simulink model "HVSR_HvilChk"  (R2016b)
settings: Solver=FixedStepDiscrete  StartTime=0.0  StopTime=10.0  FixedStep=0.02  RelTol=1e-3  EnableMultiTasking=on
undefined symbols (not defined in the file or in its folder): BCCR_cntHvilDiag_CW, bin2dec, HVSR_dcHvilPwmDutyHi_C, HVSR_dcHvilPwmDutyLo_C, HVSR_dcHvilPwmDutyNrm_C, HVSR_dcHvilPwmDutyOpl_C, HVSR_dcHvilPwmDutyOptSet_C, HVSR_dcHvilPwmDutyThres_C, HVSR_fHvilPwmFrqHi_C, HVSR_fHvilPwmFrqLo_C, HVSR_tiHvilOplErr_C, HVSR_tiHvilScbErr_C, HVSR_tiHvilScgErr_C, HVSR_uKL30ThresHi_C, HVSR_uKL30ThresLo_C
libraries: simulink x39

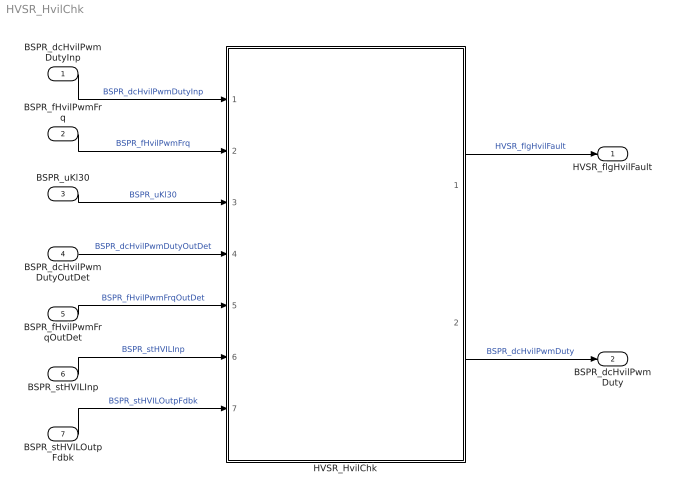
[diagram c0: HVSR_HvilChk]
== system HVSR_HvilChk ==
  BSPR_dcHvilPwmDutyInp : Inport
  BSPR_fHvilPwmFrq : Inport  Port=2
  BSPR_uKl30 : Inport  Port=3
  BSPR_dcHvilPwmDutyOutDet : Inport  Port=4
  BSPR_fHvilPwmFrqOutDet : Inport  Port=5
  BSPR_stHVILInp : Inport  Port=6
  BSPR_stHVILOutpFdbk : Inport  Port=7
  HVSR_HvilChk : Subsystem
  HVSR_flgHvilFault : Outport
  BSPR_dcHvilPwmDuty : Outport  Port=2
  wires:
  BSPR_uKl30/1 -> HVSR_HvilChk/3(BSPR_uKl30)  "BSPR_uKl30"
  BSPR_dcHvilPwmDutyInp/1 -> HVSR_HvilChk/1(BSPR_dcHvilPwmDutyInp)  "BSPR_dcHvilPwmDutyInp"
  HVSR_HvilChk/1(HVSR_flgHvilFault) -> HVSR_flgHvilFault/1  "HVSR_flgHvilFault"
  BSPR_fHvilPwmFrq/1 -> HVSR_HvilChk/2(BSPR_fHvilPwmFrq)  "BSPR_fHvilPwmFrq"
  BSPR_dcHvilPwmDutyOutDet/1 -> HVSR_HvilChk/4(BSPR_dcHvilPwmDutyOutDet)  "BSPR_dcHvilPwmDutyOutDet"
  BSPR_fHvilPwmFrqOutDet/1 -> HVSR_HvilChk/5(BSPR_fHvilPwmFrqOutDet)  "BSPR_fHvilPwmFrqOutDet"
  BSPR_stHVILInp/1 -> HVSR_HvilChk/6(BSPR_stHVILInp)  "BSPR_stHVILInp"
  BSPR_stHVILOutpFdbk/1 -> HVSR_HvilChk/7(BSPR_stHVILOutpFdbk)  "BSPR_stHVILOutpFdbk"
  HVSR_HvilChk/2(BSPR_dcHvilPwmDuty) -> BSPR_dcHvilPwmDuty/1  "BSPR_dcHvilPwmDuty"

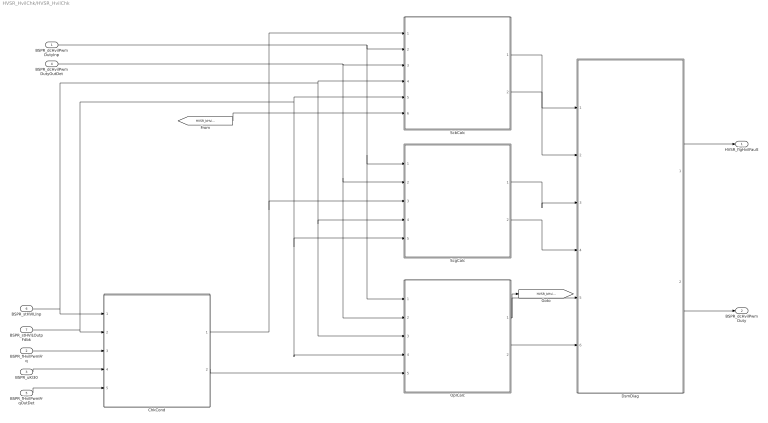
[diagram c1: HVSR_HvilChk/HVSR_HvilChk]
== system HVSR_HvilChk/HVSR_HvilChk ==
  BSPR_dcHvilPwmDutyInp : Inport
  BSPR_fHvilPwmFrq : Inport  Port=2
  BSPR_uKl30 : Inport  Port=3
  BSPR_dcHvilPwmDutyOutDet : Inport  Port=4
  BSPR_fHvilPwmFrqOutDet : Inport  Port=5
  BSPR_stHVILInp : Inport  Port=6
  BSPR_stHVILOutpFdbk : Inport  Port=7
  ChkCond : Subsystem
  DsmDiag : Subsystem
  OplCalc : Subsystem
  ScbCalc : Subsystem
  ScgCalc : Subsystem
  HVSR_flgHvilFault : Outport
  BSPR_dcHvilPwmDuty : Outport  Port=2
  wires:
  BSPR_uKl30/1 -> ChkCond/4(BSPR_uKl30)
  BSPR_dcHvilPwmDutyInp/1 -> ScgCalc/1(BSPR_dcHvilPwmDutyInp), OplCalc/1(BSPR_dcHvilPwmDutyInp), ScbCalc/2(BSPR_dcHvilPwmDutyInp)
  ScgCalc/1(HVSR_bHvilScgErrDet) -> DsmDiag/3(HVSR_bHvilScgErrDet)
  ScgCalc/2(HVSR_bHvilScgErrHeal) -> DsmDiag/4(HVSR_bHvilScgErrHeal)
  ChkCond/1(BSPR_bKl30HvilDiagCond) -> ScbCalc/1(BSPR_bKl30HvilDiagCond), ScgCalc/3(BSPR_bKl30HvilDiagCond)
  ScbCalc/1(HVSR_bHvilScbErrDet) -> DsmDiag/1(HVSR_bHvilScbErrDet)
  ScbCalc/2(HVSR_bHvilScbErrHeal) -> DsmDiag/2(HVSR_bHvilScbErrHeal)
  DsmDiag/1(HVSR_flgHvilFault) -> HVSR_flgHvilFault/1
  OplCalc/2(HVSR_bHvilOplErrHeal) -> DsmDiag/6(HVSR_bHvilOplErrHeal)
  OplCalc/1(HVSR_bHvilOplErrDet) -> [HVSR_bHvilOplErrDet], DsmDiag/5(HVSR_bHvilOplErrDet)
  BSPR_fHvilPwmFrq/1 -> ChkCond/3(BSPR_fHvilPwmFrq)
  ChkCond/2(BSPR_bHvilDiagCond) -> OplCalc/5(BSPR_bHvilDiagCond)
  BSPR_dcHvilPwmDutyOutDet/1 -> ScgCalc/2(BSPR_dcHvilPwmDutyOutDet), OplCalc/2(BSPR_dcHvilPwmDutyOutDet), ScbCalc/3(BSPR_dcHvilPwmDutyOutDet)
  BSPR_fHvilPwmFrqOutDet/1 -> ChkCond/5(BSPR_fHvilPwmFrqOutDet)
  BSPR_stHVILInp/1 -> ChkCond/1(BSPR_stHVILInp), ScgCalc/4(BSPR_stHVILInp), OplCalc/3(BSPR_stHVILInp), ScbCalc/4(BSPR_stHVILInp)
  BSPR_stHVILOutpFdbk/1 -> ChkCond/2(BSPR_stHVILOutpFdbk), ScgCalc/5(BSPR_stHVILOutpFdbk), OplCalc/4(BSPR_stHVILOutpFdbk), ScbCalc/5(BSPR_stHVILOutpFdbk)
  DsmDiag/2(BSPR_dcHvilPwmDuty) -> BSPR_dcHvilPwmDuty/1
  [HVSR_bHvilOplErrDet] -> ScbCalc/6(HVSR_bHvilOplErrDet)

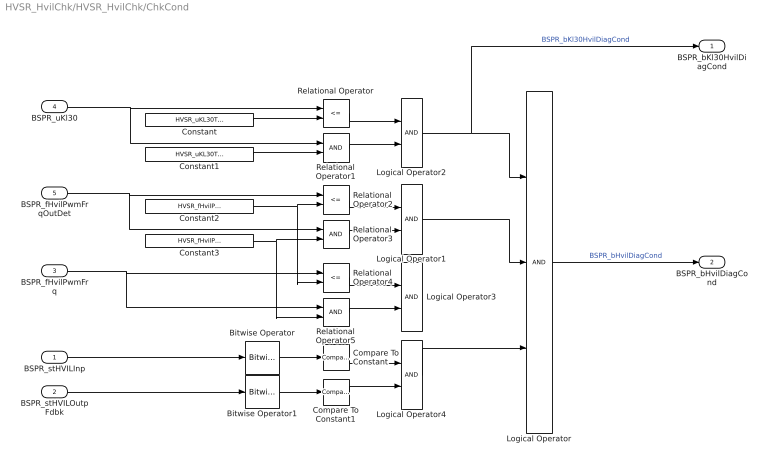
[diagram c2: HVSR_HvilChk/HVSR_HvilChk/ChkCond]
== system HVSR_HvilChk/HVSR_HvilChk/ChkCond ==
  BSPR_stHVILInp : Inport
  BSPR_stHVILOutpFdbk : Inport  Port=2
  BSPR_fHvilPwmFrq : Inport  Port=3
  BSPR_uKl30 : Inport  Port=4
  BSPR_fHvilPwmFrqOutDet : Inport  Port=5
  Bitwise Operator : simulink/Logic and Bit Operations/Bitwise Operator  logicop=AND  UseBitMask=on  BitMask=bin2dec('00010000')  BitMaskRealWorld=Stored Integer
  Bitwise Operator1 : simulink/Logic and Bit Operations/Bitwise Operator  logicop=AND  UseBitMask=on  BitMask=bin2dec('00010000')  BitMaskRealWorld=Stored Integer
  Compare To Constant : simulink/Logic and Bit Operations/Compare To Constant  relop===  const=0  OutDataTypeStr=boolean
  Compare To Constant1 : simulink/Logic and Bit Operations/Compare To Constant  relop===  const=0  OutDataTypeStr=boolean
  Constant : Constant  Value=HVSR_uKL30ThresHi_C
  Constant1 : Constant  Value=HVSR_uKL30ThresLo_C
  Constant2 : Constant  Value=HVSR_fHvilPwmFrqHi_C
  Constant3 : Constant  Value=HVSR_fHvilPwmFrqLo_C
  Logical Operator : Logic  Inputs=3  AllPortsSameDT=off  OutDataTypeStr=boolean
  Logical Operator1 : Logic  AllPortsSameDT=off  OutDataTypeStr=boolean
  Logical Operator2 : Logic  AllPortsSameDT=off  OutDataTypeStr=boolean
  Logical Operator3 : Logic  Commented=on  AllPortsSameDT=off  OutDataTypeStr=boolean
  Logical Operator4 : Logic  AllPortsSameDT=off  OutDataTypeStr=boolean
  Relational Operator : RelationalOperator  Operator=<=  OutDataTypeStr=boolean  RndMeth=Simplest
  Relational Operator1 : RelationalOperator  OutDataTypeStr=boolean  RndMeth=Simplest
  Relational Operator2 : RelationalOperator  Operator=<=  OutDataTypeStr=boolean  RndMeth=Simplest
  Relational Operator3 : RelationalOperator  OutDataTypeStr=boolean  RndMeth=Simplest
  Relational Operator4 : RelationalOperator  Commented=on  Operator=<=  OutDataTypeStr=boolean  RndMeth=Simplest
  Relational Operator5 : RelationalOperator  Commented=on  OutDataTypeStr=boolean  RndMeth=Simplest
  BSPR_bKl30HvilDiagCond : Outport
  BSPR_bHvilDiagCond : Outport  Port=2
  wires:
  BSPR_uKl30/1 -> Relational Operator/1, Relational Operator1/1
  Logical Operator/1 -> BSPR_bHvilDiagCond/1  "BSPR_bHvilDiagCond"
  Constant/1 -> Relational Operator/2
  Constant1/1 -> Relational Operator1/2
  BSPR_fHvilPwmFrqOutDet/1 -> Relational Operator2/1, Relational Operator3/1
  Relational Operator/1 -> Logical Operator2/1
  Relational Operator1/1 -> Logical Operator2/2
  Logical Operator2/1 -> BSPR_bKl30HvilDiagCond/1, Logical Operator/1  "BSPR_bKl30HvilDiagCond"
  BSPR_fHvilPwmFrq/1 -> Relational Operator5/1, Relational Operator4/1
  Constant2/1 -> Relational Operator4/2, Relational Operator2/2
  Constant3/1 -> Relational Operator5/2, Relational Operator3/2
  Relational Operator4/1 -> Logical Operator3/1
  Relational Operator5/1 -> Logical Operator3/2
  Relational Operator2/1 -> Logical Operator1/1
  Relational Operator3/1 -> Logical Operator1/2
  Logical Operator1/1 -> Logical Operator/2
  Logical Operator3/1 -> ?
  BSPR_stHVILInp/1 -> Bitwise Operator/1
  BSPR_stHVILOutpFdbk/1 -> Bitwise Operator1/1
  Bitwise Operator/1 -> Compare To Constant/1
  Bitwise Operator1/1 -> Compare To Constant1/1
  Compare To Constant/1 -> Logical Operator4/1
  Compare To Constant1/1 -> Logical Operator4/2
  Logical Operator4/1 -> Logical Operator/3

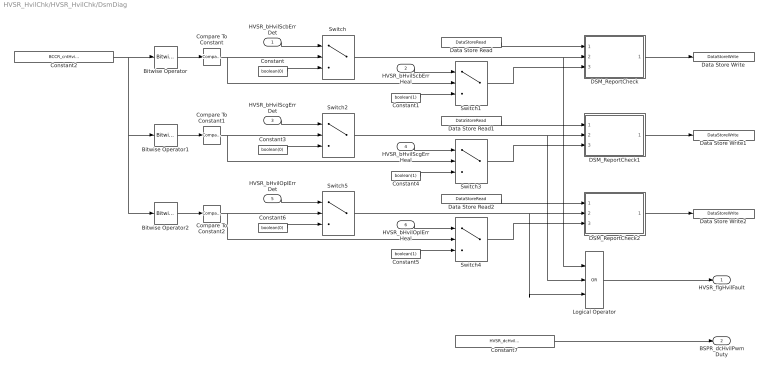
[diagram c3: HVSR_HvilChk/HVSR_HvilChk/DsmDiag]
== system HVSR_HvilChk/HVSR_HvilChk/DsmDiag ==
  HVSR_bHvilScbErrDet : Inport
  HVSR_bHvilScbErrHeal : Inport  Port=2
  HVSR_bHvilScgErrDet : Inport  Port=3
  HVSR_bHvilScgErrHeal : Inport  Port=4
  HVSR_bHvilOplErrDet : Inport  Port=5
  HVSR_bHvilOplErrHeal : Inport  Port=6
  Bitwise Operator : simulink/Logic and Bit Operations/Bitwise Operator  logicop=AND  UseBitMask=on  BitMask=bin2dec('00000001')  BitMaskRealWorld=Stored Integer
  Bitwise Operator1 : simulink/Logic and Bit Operations/Bitwise Operator  logicop=AND  UseBitMask=on  BitMask=bin2dec('00000010')  BitMaskRealWorld=Stored Integer
  Bitwise Operator2 : simulink/Logic and Bit Operations/Bitwise Operator  logicop=AND  UseBitMask=on  BitMask=bin2dec('00000100')  BitMaskRealWorld=Stored Integer
  Compare To Constant : simulink/Logic and Bit Operations/Compare To Constant  relop===  const=1  OutDataTypeStr=boolean
  Compare To Constant1 : simulink/Logic and Bit Operations/Compare To Constant  relop===  const=2  OutDataTypeStr=boolean
  Compare To Constant2 : simulink/Logic and Bit Operations/Compare To Constant  relop===  const=4  OutDataTypeStr=boolean
  Constant : Constant  Value=boolean(0)  OutDataTypeStr=boolean
  Constant1 : Constant  Value=boolean(1)  OutDataTypeStr=boolean
  Constant2 : Constant  Value=BCCR_cntHvilDiag_CW
  Constant3 : Constant  Value=boolean(0)  OutDataTypeStr=boolean
  Constant4 : Constant  Value=boolean(1)  OutDataTypeStr=boolean
  Constant5 : Constant  Value=boolean(1)  OutDataTypeStr=boolean
  Constant6 : Constant  Value=boolean(0)  OutDataTypeStr=boolean
  Constant7 : Constant  Value=HVSR_dcHvilPwmDutyOptSet_C
  DSM_ReportCheck : Subsystem  TreatAsAtomicUnit=on  RTWFcnName=DSM_ReportCheck  RTWFileName=SrvLib
  DSM_ReportCheck1 : Subsystem  TreatAsAtomicUnit=on  RTWFcnName=DSM_ReportCheck  RTWFileName=SrvLib
  DSM_ReportCheck2 : Subsystem  TreatAsAtomicUnit=on  RTWFcnName=DSM_ReportCheck  RTWFileName=SrvLib
  Data Store Read : DataStoreRead  DataStoreName=DFC_HvilMax
  Data Store Read1 : DataStoreRead  DataStoreName=DFC_HvilMin
  Data Store Read2 : DataStoreRead  DataStoreName=DFC_HvilSig
  Data Store Write : DataStoreWrite  DataStoreName=DFC_HvilMax
  Data Store Write1 : DataStoreWrite  DataStoreName=DFC_HvilMin
  Data Store Write2 : DataStoreWrite  DataStoreName=DFC_HvilSig
  Logical Operator : Logic  Operator=OR  Inputs=3  AllPortsSameDT=off  OutDataTypeStr=boolean
  Switch{,1..5} (6 alike) : Switch  Criteria=u2 > Threshold
  HVSR_flgHvilFault : Outport
  BSPR_dcHvilPwmDuty : Outport  Port=2
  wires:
  Data Store Read1/1 -> DSM_ReportCheck1/1(Dfc_id_nv)
  DSM_ReportCheck2/1(Dfc_id) -> Data Store Write2/1
  Data Store Read/1 -> DSM_ReportCheck/1(Dfc_id_nv)
  Data Store Read2/1 -> DSM_ReportCheck2/1(Dfc_id_nv)
  DSM_ReportCheck1/1(Dfc_id) -> Data Store Write1/1
  DSM_ReportCheck/1(Dfc_id) -> Data Store Write/1
  Constant/1 -> Switch/3
  Constant1/1 -> Switch1/3
  Switch1/1 -> DSM_ReportCheck/3(Heal)
  Switch/1 -> DSM_ReportCheck/2(Err), Logical Operator/1
  Constant2/1 -> Bitwise Operator2/1, Bitwise Operator1/1, Bitwise Operator/1
  Bitwise Operator/1 -> Compare To Constant/1
  Compare To Constant/1 -> Switch1/2, Switch/2
  Constant3/1 -> Switch2/3
  Constant4/1 -> Switch3/3
  Switch3/1 -> DSM_ReportCheck1/3(Heal)
  Switch2/1 -> DSM_ReportCheck1/2(Err), Logical Operator/2
  Bitwise Operator1/1 -> Compare To Constant1/1
  Compare To Constant1/1 -> Switch3/2, Switch2/2
  Constant5/1 -> Switch4/3
  Switch4/1 -> DSM_ReportCheck2/3(Heal)
  Constant6/1 -> Switch5/3
  Switch5/1 -> DSM_ReportCheck2/2(Err), Logical Operator/3
  HVSR_bHvilOplErrHeal/1 -> Switch4/1
  HVSR_bHvilOplErrDet/1 -> Switch5/1
  Bitwise Operator2/1 -> Compare To Constant2/1
  Compare To Constant2/1 -> Switch4/2, Switch5/2
  HVSR_bHvilScgErrHeal/1 -> Switch3/1
  HVSR_bHvilScgErrDet/1 -> Switch2/1
  HVSR_bHvilScbErrDet/1 -> Switch/1
  HVSR_bHvilScbErrHeal/1 -> Switch1/1
  Logical Operator/1 -> HVSR_flgHvilFault/1
  Constant7/1 -> BSPR_dcHvilPwmDuty/1

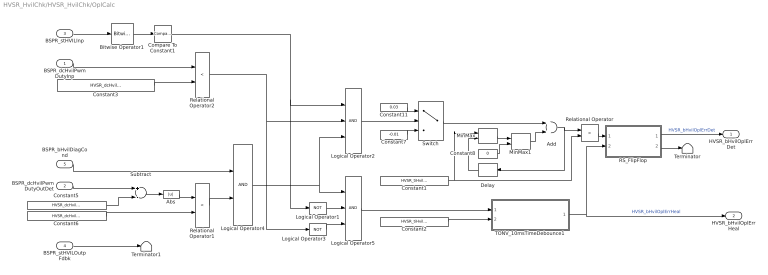
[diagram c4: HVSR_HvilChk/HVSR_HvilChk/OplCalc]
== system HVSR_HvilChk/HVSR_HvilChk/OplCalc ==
  BSPR_dcHvilPwmDutyInp : Inport
  BSPR_dcHvilPwmDutyOutDet : Inport  Port=2
  BSPR_stHVILInp : Inport  Port=3
  BSPR_stHVILOutpFdbk : Inport  Port=4
  BSPR_bHvilDiagCond : Inport  Port=5
  Abs : Abs
  Add : Sum
  Bitwise Operator1 : simulink/Logic and Bit Operations/Bitwise Operator  logicop=AND  UseBitMask=on  BitMask=bin2dec('00001000')  BitMaskRealWorld=Stored Integer
  Compare To Constant1 : simulink/Logic and Bit Operations/Compare To Constant  relop===  const=8  OutDataTypeStr=boolean
  Constant1 : Constant  Value=HVSR_tiHvilOplErr_C
  Constant11 : Constant  Value=0.03  OutDataTypeStr=single
  Constant2 : Constant  Value=HVSR_tiHvilOplErr_C
  Constant3 : Constant  Value=HVSR_dcHvilPwmDutyOpl_C
  Constant5 : Constant  Value=HVSR_dcHvilPwmDutyNrm_C
  Constant6 : Constant  Value=HVSR_dcHvilPwmDutyThres_C
  Constant7 : Constant  Value=-0.01  OutDataTypeStr=single
  Constant8 : Constant  Value=0  OutDataTypeStr=single
  Delay : Delay  DelayLength=1  InitialCondition=0
  Logical Operator1 : Logic  Operator=NOT  AllPortsSameDT=off  OutDataTypeStr=boolean
  Logical Operator2 : Logic  Inputs=3  AllPortsSameDT=off  OutDataTypeStr=boolean
  Logical Operator3 : Logic  Operator=NOT  AllPortsSameDT=off  OutDataTypeStr=boolean
  Logical Operator4 : Logic  AllPortsSameDT=off  OutDataTypeStr=boolean
  Logical Operator5 : Logic  Inputs=3  AllPortsSameDT=off  OutDataTypeStr=boolean
  MinMax : MinMax  Inputs=2
  MinMax1 : MinMax  Function=max  Inputs=2
  RS_FlipFlop : Subsystem
  Relational Operator : RelationalOperator  Operator=>  OutDataTypeStr=boolean  RndMeth=Simplest
  Relational Operator1 : RelationalOperator  Operator=<  OutDataTypeStr=boolean  RndMeth=Simplest
  Relational Operator2 : RelationalOperator  Operator=<  OutDataTypeStr=boolean  RndMeth=Simplest
  Subtract : Sum  Inputs=+-
  Switch : Switch  Criteria=u2 ~= 0
  TONV_10msTimeDebounce1 : Subsystem  TreatAsAtomicUnit=on  RTWFcnName=TONV_10msTimeDebounce  RTWFileName=SrvLib
  Terminator : Terminator
  Terminator1 : Terminator
  HVSR_bHvilOplErrDet : Outport
  HVSR_bHvilOplErrHeal : Outport  Port=2
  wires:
  BSPR_bHvilDiagCond/1 -> Logical Operator4/1
  Logical Operator5/1 -> TONV_10msTimeDebounce1/1(u)
  Constant2/1 -> TONV_10msTimeDebounce1/2(T)
  Subtract/1 -> Abs/1
  Constant5/1 -> Subtract/2
  Abs/1 -> Relational Operator1/1
  Constant6/1 -> Relational Operator1/2
  Relational Operator1/1 -> Logical Operator4/2
  Relational Operator2/1 -> Logical Operator2/2, Logical Operator3/1
  MinMax1/1 -> Add/2
  Constant1/1 -> Relational Operator/2, MinMax/1
  Delay/1 -> MinMax/2
  Switch/1 -> Add/1
  Add/1 -> Delay/1, Relational Operator/1
  Constant7/1 -> Switch/3
  Constant11/1 -> Switch/1
  MinMax/1 -> MinMax1/1
  Constant8/1 -> MinMax1/2
  Logical Operator2/1 -> Switch/2
  Relational Operator/1 -> RS_FlipFlop/1(S)
  Logical Operator3/1 -> Logical Operator5/3
  Logical Operator4/1 -> Logical Operator5/1, Logical Operator2/3
  TONV_10msTimeDebounce1/1(y) -> RS_FlipFlop/2(R), HVSR_bHvilOplErrHeal/1  "HVSR_bHvilOplErrHeal"
  RS_FlipFlop/2(!Q) -> Terminator/1
  RS_FlipFlop/1(Q) -> HVSR_bHvilOplErrDet/1  "HVSR_bHvilOplErrDet"
  BSPR_dcHvilPwmDutyOutDet/1 -> Subtract/1
  BSPR_dcHvilPwmDutyInp/1 -> Relational Operator2/1
  Constant3/1 -> Relational Operator2/2
  Bitwise Operator1/1 -> Compare To Constant1/1
  BSPR_stHVILInp/1 -> Bitwise Operator1/1
  BSPR_stHVILOutpFdbk/1 -> Terminator1/1
  Compare To Constant1/1 -> Logical Operator2/1, Logical Operator1/1
  Logical Operator1/1 -> Logical Operator5/2

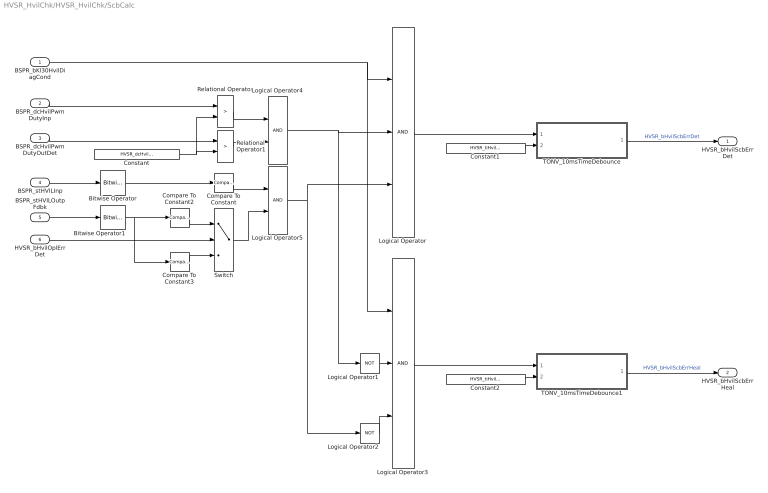
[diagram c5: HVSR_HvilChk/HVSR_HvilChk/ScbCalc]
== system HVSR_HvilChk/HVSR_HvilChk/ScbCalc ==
  BSPR_bKl30HvilDiagCond : Inport
  BSPR_dcHvilPwmDutyInp : Inport  Port=2
  BSPR_dcHvilPwmDutyOutDet : Inport  Port=3
  BSPR_stHVILInp : Inport  Port=4
  BSPR_stHVILOutpFdbk : Inport  Port=5
  HVSR_bHvilOplErrDet : Inport  Port=6
  Bitwise Operator : simulink/Logic and Bit Operations/Bitwise Operator  logicop=AND  UseBitMask=on  BitMask=bin2dec('00001001')  BitMaskRealWorld=Stored Integer
  Bitwise Operator1 : simulink/Logic and Bit Operations/Bitwise Operator  logicop=AND  UseBitMask=on  BitMask=bin2dec('00001001')  BitMaskRealWorld=Stored Integer
  Compare To Constant : simulink/Logic and Bit Operations/Compare To Constant  relop===  const=9  OutDataTypeStr=boolean
  Compare To Constant2 : simulink/Logic and Bit Operations/Compare To Constant  relop===  const=8  OutDataTypeStr=boolean
  Compare To Constant3 : simulink/Logic and Bit Operations/Compare To Constant  relop===  const=9  OutDataTypeStr=boolean
  Constant : Constant  Value=HVSR_dcHvilPwmDutyHi_C
  Constant1 : Constant  Value=HVSR_tiHvilScbErr_C
  Constant2 : Constant  Value=HVSR_tiHvilScbErr_C
  Logical Operator : Logic  Inputs=3  AllPortsSameDT=off  OutDataTypeStr=boolean
  Logical Operator1 : Logic  Operator=NOT  AllPortsSameDT=off  OutDataTypeStr=boolean
  Logical Operator2 : Logic  Operator=NOT  AllPortsSameDT=off  OutDataTypeStr=boolean
  Logical Operator3 : Logic  Inputs=3  AllPortsSameDT=off  OutDataTypeStr=boolean
  Logical Operator4 : Logic  AllPortsSameDT=off  OutDataTypeStr=boolean
  Logical Operator5 : Logic  AllPortsSameDT=off  OutDataTypeStr=boolean
  Relational Operator : RelationalOperator  Operator=>  OutDataTypeStr=boolean  RndMeth=Simplest
  Relational Operator1 : RelationalOperator  Operator=>  OutDataTypeStr=boolean  RndMeth=Simplest
  Switch : Switch  Criteria=u2 ~= 0
  TONV_10msTimeDebounce : Subsystem  TreatAsAtomicUnit=on  RTWFcnName=TONV_10msTimeDebounce  RTWFileName=SrvLib
  TONV_10msTimeDebounce1 : Subsystem  TreatAsAtomicUnit=on  RTWFcnName=TONV_10msTimeDebounce  RTWFileName=SrvLib
  HVSR_bHvilScbErrDet : Outport
  HVSR_bHvilScbErrHeal : Outport  Port=2
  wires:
  Logical Operator2/1 -> Logical Operator3/3
  TONV_10msTimeDebounce1/1(y) -> HVSR_bHvilScbErrHeal/1  "HVSR_bHvilScbErrHeal"
  Logical Operator3/1 -> TONV_10msTimeDebounce1/1(u)
  Constant2/1 -> TONV_10msTimeDebounce1/2(T)
  BSPR_bKl30HvilDiagCond/1 -> Logical Operator/1, Logical Operator3/1
  Constant1/1 -> TONV_10msTimeDebounce/2(T)
  Logical Operator/1 -> TONV_10msTimeDebounce/1(u)
  Constant/1 -> Relational Operator/2, Relational Operator1/2
  BSPR_dcHvilPwmDutyInp/1 -> Relational Operator/1
  TONV_10msTimeDebounce/1(y) -> HVSR_bHvilScbErrDet/1  "HVSR_bHvilScbErrDet"
  BSPR_dcHvilPwmDutyOutDet/1 -> Relational Operator1/1
  Logical Operator1/1 -> Logical Operator3/2
  Bitwise Operator/1 -> Compare To Constant/1
  BSPR_stHVILInp/1 -> Bitwise Operator/1
  BSPR_stHVILOutpFdbk/1 -> Bitwise Operator1/1
  Relational Operator1/1 -> Logical Operator4/2
  Relational Operator/1 -> Logical Operator4/1
  Logical Operator4/1 -> Logical Operator/2, Logical Operator1/1
  Compare To Constant/1 -> Logical Operator5/1
  Logical Operator5/1 -> Logical Operator/3, Logical Operator2/1
  HVSR_bHvilOplErrDet/1 -> Switch/2
  Bitwise Operator1/1 -> Compare To Constant2/1, Compare To Constant3/1
  Compare To Constant2/1 -> Switch/1
  Compare To Constant3/1 -> Switch/3
  Switch/1 -> Logical Operator5/2

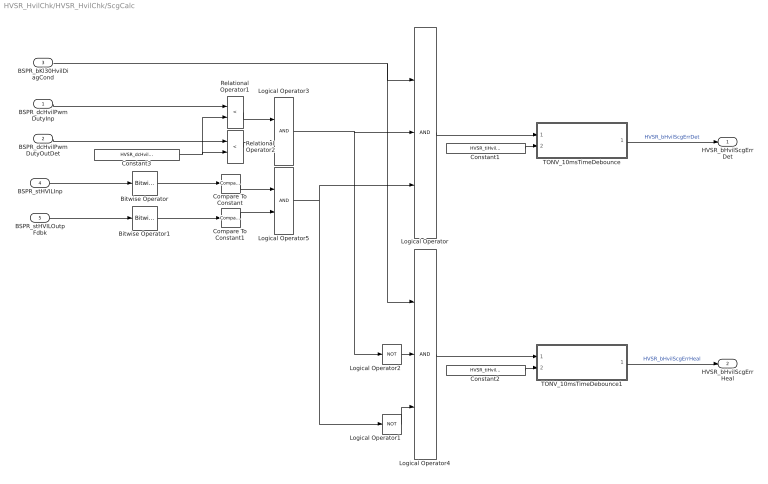
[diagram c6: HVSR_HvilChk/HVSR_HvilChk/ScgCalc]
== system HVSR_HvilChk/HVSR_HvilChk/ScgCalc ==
  BSPR_dcHvilPwmDutyInp : Inport
  BSPR_dcHvilPwmDutyOutDet : Inport  Port=2
  BSPR_bKl30HvilDiagCond : Inport  Port=3
  BSPR_stHVILInp : Inport  Port=4
  BSPR_stHVILOutpFdbk : Inport  Port=5
  Bitwise Operator : simulink/Logic and Bit Operations/Bitwise Operator  logicop=AND  UseBitMask=on  BitMask=bin2dec('00001001')  BitMaskRealWorld=Stored Integer
  Bitwise Operator1 : simulink/Logic and Bit Operations/Bitwise Operator  logicop=AND  UseBitMask=on  BitMask=bin2dec('00001001')  BitMaskRealWorld=Stored Integer
  Compare To Constant : simulink/Logic and Bit Operations/Compare To Constant  relop===  const=8  OutDataTypeStr=boolean
  Compare To Constant1 : simulink/Logic and Bit Operations/Compare To Constant  relop===  const=8  OutDataTypeStr=boolean
  Constant1 : Constant  Value=HVSR_tiHvilScgErr_C
  Constant2 : Constant  Value=HVSR_tiHvilScgErr_C
  Constant3 : Constant  Value=HVSR_dcHvilPwmDutyLo_C
  Logical Operator : Logic  Inputs=3  AllPortsSameDT=off  OutDataTypeStr=boolean
  Logical Operator1 : Logic  Operator=NOT  AllPortsSameDT=off  OutDataTypeStr=boolean
  Logical Operator2 : Logic  Operator=NOT  AllPortsSameDT=off  OutDataTypeStr=boolean
  Logical Operator3 : Logic  AllPortsSameDT=off  OutDataTypeStr=boolean
  Logical Operator4 : Logic  Inputs=3  AllPortsSameDT=off  OutDataTypeStr=boolean
  Logical Operator5 : Logic  AllPortsSameDT=off  OutDataTypeStr=boolean
  Relational Operator1 : RelationalOperator  Operator=<  OutDataTypeStr=boolean  RndMeth=Simplest
  Relational Operator2 : RelationalOperator  Operator=<  OutDataTypeStr=boolean  RndMeth=Simplest
  TONV_10msTimeDebounce : Subsystem  TreatAsAtomicUnit=on  RTWFcnName=TONV_10msTimeDebounce  RTWFileName=SrvLib
  TONV_10msTimeDebounce1 : Subsystem  TreatAsAtomicUnit=on  RTWFcnName=TONV_10msTimeDebounce  RTWFileName=SrvLib
  HVSR_bHvilScgErrDet : Outport
  HVSR_bHvilScgErrHeal : Outport  Port=2
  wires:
  TONV_10msTimeDebounce/1(y) -> HVSR_bHvilScgErrDet/1  "HVSR_bHvilScgErrDet"
  Constant1/1 -> TONV_10msTimeDebounce/2(T)
  Constant2/1 -> TONV_10msTimeDebounce1/2(T)
  TONV_10msTimeDebounce1/1(y) -> HVSR_bHvilScgErrHeal/1  "HVSR_bHvilScgErrHeal"
  Logical Operator4/1 -> TONV_10msTimeDebounce1/1(u)
  Logical Operator/1 -> TONV_10msTimeDebounce/1(u)
  Constant3/1 -> Relational Operator1/2, Relational Operator2/2
  BSPR_bKl30HvilDiagCond/1 -> Logical Operator4/1, Logical Operator/1
  BSPR_dcHvilPwmDutyInp/1 -> Relational Operator1/1
  Logical Operator2/1 -> Logical Operator4/2
  BSPR_dcHvilPwmDutyOutDet/1 -> Relational Operator2/1
  Logical Operator1/1 -> Logical Operator4/3
  Bitwise Operator/1 -> Compare To Constant/1
  Bitwise Operator1/1 -> Compare To Constant1/1
  Compare To Constant/1 -> Logical Operator5/1
  Compare To Constant1/1 -> Logical Operator5/2
  BSPR_stHVILInp/1 -> Bitwise Operator/1
  BSPR_stHVILOutpFdbk/1 -> Bitwise Operator1/1
  Relational Operator1/1 -> Logical Operator3/1
  Relational Operator2/1 -> Logical Operator3/2
  Logical Operator3/1 -> Logical Operator2/1, Logical Operator/2
  Logical Operator5/1 -> Logical Operator1/1, Logical Operator/3

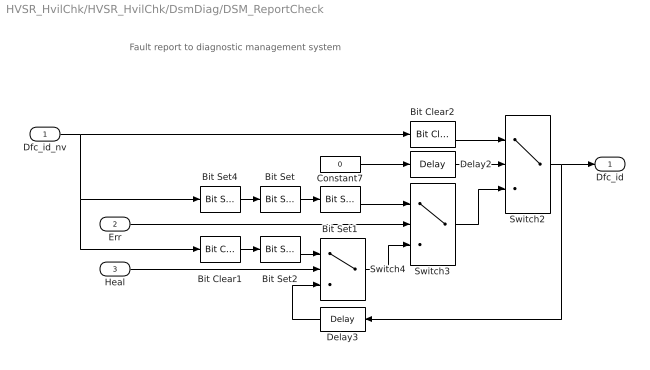
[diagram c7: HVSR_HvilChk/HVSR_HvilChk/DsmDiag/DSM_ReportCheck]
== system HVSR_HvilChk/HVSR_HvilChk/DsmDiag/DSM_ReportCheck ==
  note: Fault report to diagnostic management system
  Dfc_id_nv : Inport  OutDataTypeStr=uint8
  Err : Inport  Port=2
  Heal : Inport  Port=3
  Bit Clear1 : simulink/Logic and Bit Operations/Bit Clear  iBit=4
  Bit Clear2 : simulink/Logic and Bit Operations/Bit Clear  iBit=3
  Bit Set : simulink/Logic and Bit Operations/Bit Set  iBit=4
  Bit Set1 : simulink/Logic and Bit Operations/Bit Set  iBit=3
  Bit Set2 : simulink/Logic and Bit Operations/Bit Set  iBit=3
  Bit Set4 : simulink/Logic and Bit Operations/Bit Set  iBit=7
  Constant7 : Constant  Value=0  OutDataTypeStr=boolean
  Delay2 : Delay  DelayLength=1  InitialCondition=1
  Delay3 : Delay  DelayLength=1  InitialCondition=0
  Switch2 : Switch  Criteria=u2 ~= 0
  Switch3 : Switch  Criteria=u2 ~= 0
  Switch4 : Switch  Criteria=u2 ~= 0
  Dfc_id : Outport  OutDataTypeStr=uint8
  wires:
  Dfc_id_nv/1 -> Bit Clear2/1, Bit Set4/1, Bit Clear1/1
  Bit Set4/1 -> Bit Set/1
  Constant7/1 -> Delay2/1
  Delay2/1 -> Switch2/2
  Switch3/1 -> Switch2/3
  Bit Clear2/1 -> Switch2/1
  Switch2/1 -> Delay3/1, Dfc_id/1
  Bit Set1/1 -> Switch3/1
  Bit Set/1 -> Bit Set1/1
  Switch4/1 -> Switch3/3
  Err/1 -> Switch3/2
  Bit Set2/1 -> Switch4/1
  Bit Clear1/1 -> Bit Set2/1
  Delay3/1 -> Switch4/3
  Heal/1 -> Switch4/2

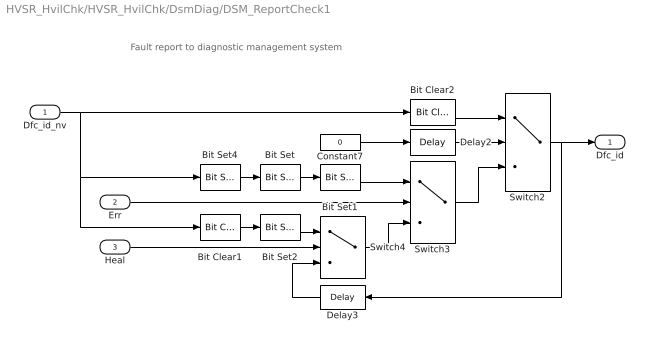
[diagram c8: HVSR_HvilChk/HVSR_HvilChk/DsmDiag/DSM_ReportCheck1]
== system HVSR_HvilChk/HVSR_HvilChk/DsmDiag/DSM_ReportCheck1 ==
  note: Fault report to diagnostic management system
  Dfc_id_nv : Inport  OutDataTypeStr=uint8
  Err : Inport  Port=2
  Heal : Inport  Port=3
  Bit Clear1 : simulink/Logic and Bit Operations/Bit Clear  iBit=4
  Bit Clear2 : simulink/Logic and Bit Operations/Bit Clear  iBit=3
  Bit Set : simulink/Logic and Bit Operations/Bit Set  iBit=4
  Bit Set1 : simulink/Logic and Bit Operations/Bit Set  iBit=3
  Bit Set2 : simulink/Logic and Bit Operations/Bit Set  iBit=3
  Bit Set4 : simulink/Logic and Bit Operations/Bit Set  iBit=7
  Constant7 : Constant  Value=0  OutDataTypeStr=boolean
  Delay2 : Delay  DelayLength=1  InitialCondition=1
  Delay3 : Delay  DelayLength=1  InitialCondition=0
  Switch2 : Switch  Criteria=u2 ~= 0
  Switch3 : Switch  Criteria=u2 ~= 0
  Switch4 : Switch  Criteria=u2 ~= 0
  Dfc_id : Outport  OutDataTypeStr=uint8
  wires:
  Heal/1 -> Switch4/2
  Delay3/1 -> Switch4/3
  Bit Clear1/1 -> Bit Set2/1
  Bit Set2/1 -> Switch4/1
  Err/1 -> Switch3/2
  Switch4/1 -> Switch3/3
  Bit Set/1 -> Bit Set1/1
  Bit Set1/1 -> Switch3/1
  Switch2/1 -> Dfc_id/1, Delay3/1
  Bit Clear2/1 -> Switch2/1
  Switch3/1 -> Switch2/3
  Delay2/1 -> Switch2/2
  Constant7/1 -> Delay2/1
  Bit Set4/1 -> Bit Set/1
  Dfc_id_nv/1 -> Bit Clear1/1, Bit Set4/1, Bit Clear2/1

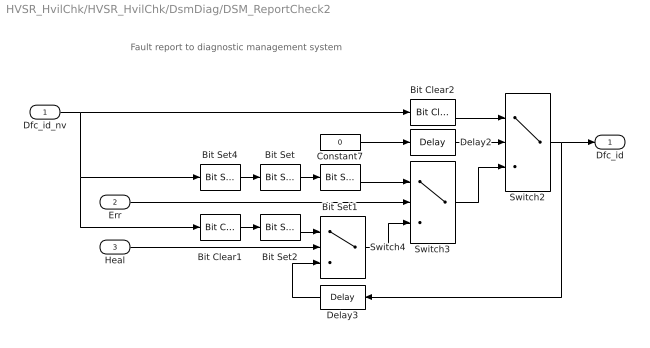
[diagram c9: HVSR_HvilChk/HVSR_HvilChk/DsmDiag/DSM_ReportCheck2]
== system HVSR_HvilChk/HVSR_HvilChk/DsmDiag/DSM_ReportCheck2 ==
  note: Fault report to diagnostic management system
  Dfc_id_nv : Inport  OutDataTypeStr=uint8
  Err : Inport  Port=2
  Heal : Inport  Port=3
  Bit Clear1 : simulink/Logic and Bit Operations/Bit Clear  iBit=4
  Bit Clear2 : simulink/Logic and Bit Operations/Bit Clear  iBit=3
  Bit Set : simulink/Logic and Bit Operations/Bit Set  iBit=4
  Bit Set1 : simulink/Logic and Bit Operations/Bit Set  iBit=3
  Bit Set2 : simulink/Logic and Bit Operations/Bit Set  iBit=3
  Bit Set4 : simulink/Logic and Bit Operations/Bit Set  iBit=7
  Constant7 : Constant  Value=0  OutDataTypeStr=boolean
  Delay2 : Delay  DelayLength=1  InitialCondition=1
  Delay3 : Delay  DelayLength=1  InitialCondition=0
  Switch2 : Switch  Criteria=u2 ~= 0
  Switch3 : Switch  Criteria=u2 ~= 0
  Switch4 : Switch  Criteria=u2 ~= 0
  Dfc_id : Outport  OutDataTypeStr=uint8
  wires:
  Dfc_id_nv/1 -> Bit Clear2/1, Bit Set4/1, Bit Clear1/1
  Bit Set4/1 -> Bit Set/1
  Constant7/1 -> Delay2/1
  Delay2/1 -> Switch2/2
  Switch3/1 -> Switch2/3
  Bit Clear2/1 -> Switch2/1
  Switch2/1 -> Delay3/1, Dfc_id/1
  Bit Set1/1 -> Switch3/1
  Bit Set/1 -> Bit Set1/1
  Switch4/1 -> Switch3/3
  Err/1 -> Switch3/2
  Bit Set2/1 -> Switch4/1
  Bit Clear1/1 -> Bit Set2/1
  Delay3/1 -> Switch4/3
  Heal/1 -> Switch4/2

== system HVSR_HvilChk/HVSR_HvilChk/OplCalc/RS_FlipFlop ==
  S : Inport  OutDataTypeStr=boolean
  R : Inport  Port=2  OutDataTypeStr=boolean
  RS : Stateflow chart  TreatAsAtomicUnit=on
  Q : Outport  OutDataTypeStr=boolean
  !Q : Outport  Port=2  OutDataTypeStr=boolean
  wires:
  R/1 -> RS/2(R)
  S/1 -> RS/1(S)
  RS/2(nQ) -> !Q/1
  RS/1(Q) -> Q/1

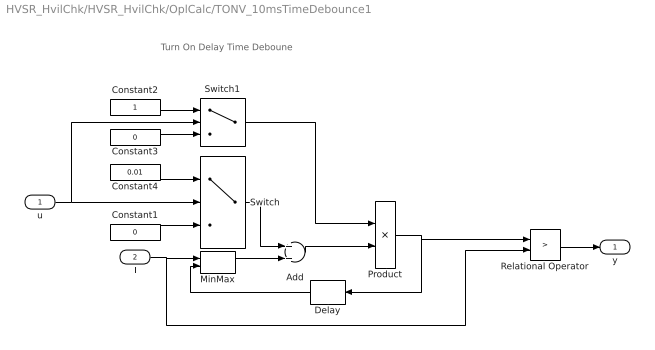
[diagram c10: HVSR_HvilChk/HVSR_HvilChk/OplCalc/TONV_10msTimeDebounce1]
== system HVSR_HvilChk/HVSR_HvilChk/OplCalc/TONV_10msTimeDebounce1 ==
  note: Turn On Delay Time Deboune
  u : Inport
  T : Inport  Port=2
  Add : Sum
  Constant1 : Constant  Value=0  OutDataTypeStr=single
  Constant2 : Constant  OutDataTypeStr=uint8
  Constant3 : Constant  Value=0  OutDataTypeStr=uint8
  Constant4 : Constant  Value=0.01  OutDataTypeStr=single
  Delay : Delay  DelayLength=1  InitialCondition=0
  MinMax : MinMax  Inputs=2
  Product : Product  OutMin=[0]  OutMax=[65535]  OutDataTypeStr=single
  Relational Operator : RelationalOperator  Operator=>  OutDataTypeStr=boolean  RndMeth=Simplest
  Switch : Switch  Criteria=u2 ~= 0
  Switch1 : Switch  Criteria=u2 ~= 0
  y : Outport
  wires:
  Switch1/1 -> Product/1
  Constant3/1 -> Switch1/3
  Constant2/1 -> Switch1/1
  u/1 -> Switch1/2, Switch/2
  Constant4/1 -> Switch/1
  Constant1/1 -> Switch/3
  Add/1 -> Product/2
  Product/1 -> Relational Operator/1, Delay/1
  Switch/1 -> Add/1
  Delay/1 -> MinMax/2
  Relational Operator/1 -> y/1
  T/1 -> MinMax/1, Relational Operator/2
  MinMax/1 -> Add/2

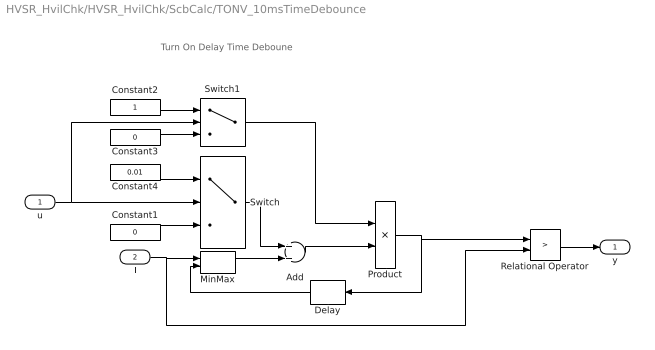
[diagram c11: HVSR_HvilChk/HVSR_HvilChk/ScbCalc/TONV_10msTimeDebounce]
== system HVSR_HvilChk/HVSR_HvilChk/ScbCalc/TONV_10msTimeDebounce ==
  note: Turn On Delay Time Deboune
  u : Inport
  T : Inport  Port=2
  Add : Sum
  Constant1 : Constant  Value=0  OutDataTypeStr=single
  Constant2 : Constant  OutDataTypeStr=uint8
  Constant3 : Constant  Value=0  OutDataTypeStr=uint8
  Constant4 : Constant  Value=0.01  OutDataTypeStr=single
  Delay : Delay  DelayLength=1  InitialCondition=0
  MinMax : MinMax  Inputs=2
  Product : Product  OutMin=[0]  OutMax=[65535]  OutDataTypeStr=single
  Relational Operator : RelationalOperator  Operator=>  OutDataTypeStr=boolean  RndMeth=Simplest
  Switch : Switch  Criteria=u2 ~= 0
  Switch1 : Switch  Criteria=u2 ~= 0
  y : Outport
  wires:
  Switch1/1 -> Product/1
  Constant3/1 -> Switch1/3
  Constant2/1 -> Switch1/1
  u/1 -> Switch1/2, Switch/2
  Constant4/1 -> Switch/1
  Constant1/1 -> Switch/3
  Add/1 -> Product/2
  Product/1 -> Relational Operator/1, Delay/1
  Switch/1 -> Add/1
  Delay/1 -> MinMax/2
  Relational Operator/1 -> y/1
  T/1 -> MinMax/1, Relational Operator/2
  MinMax/1 -> Add/2

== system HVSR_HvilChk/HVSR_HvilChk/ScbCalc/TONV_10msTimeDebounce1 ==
  note: Turn On Delay Time Deboune
  u : Inport
  T : Inport  Port=2
  Add : Sum
  Constant1 : Constant  Value=0  OutDataTypeStr=single
  Constant2 : Constant  OutDataTypeStr=uint8
  Constant3 : Constant  Value=0  OutDataTypeStr=uint8
  Constant4 : Constant  Value=0.01  OutDataTypeStr=single
  Delay : Delay  DelayLength=1  InitialCondition=0
  MinMax : MinMax  Inputs=2
  Product : Product  OutMin=[0]  OutMax=[65535]  OutDataTypeStr=single
  Relational Operator : RelationalOperator  Operator=>  OutDataTypeStr=boolean  RndMeth=Simplest
  Switch : Switch  Criteria=u2 ~= 0
  Switch1 : Switch  Criteria=u2 ~= 0
  y : Outport
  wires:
  MinMax/1 -> Add/2
  T/1 -> Relational Operator/2, MinMax/1
  Relational Operator/1 -> y/1
  Delay/1 -> MinMax/2
  Switch/1 -> Add/1
  Product/1 -> Delay/1, Relational Operator/1
  Add/1 -> Product/2
  Constant1/1 -> Switch/3
  Constant4/1 -> Switch/1
  u/1 -> Switch/2, Switch1/2
  Constant2/1 -> Switch1/1
  Constant3/1 -> Switch1/3
  Switch1/1 -> Product/1

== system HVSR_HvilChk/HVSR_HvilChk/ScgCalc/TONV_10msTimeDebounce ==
  note: Turn On Delay Time Deboune
  u : Inport
  T : Inport  Port=2
  Add : Sum
  Constant1 : Constant  Value=0  OutDataTypeStr=single
  Constant2 : Constant  OutDataTypeStr=uint8
  Constant3 : Constant  Value=0  OutDataTypeStr=uint8
  Constant4 : Constant  Value=0.01  OutDataTypeStr=single
  Delay : Delay  DelayLength=1  InitialCondition=0
  MinMax : MinMax  Inputs=2
  Product : Product  OutMin=[0]  OutMax=[65535]  OutDataTypeStr=single
  Relational Operator : RelationalOperator  Operator=>  OutDataTypeStr=boolean  RndMeth=Simplest
  Switch : Switch  Criteria=u2 ~= 0
  Switch1 : Switch  Criteria=u2 ~= 0
  y : Outport
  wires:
  MinMax/1 -> Add/2
  T/1 -> Relational Operator/2, MinMax/1
  Relational Operator/1 -> y/1
  Delay/1 -> MinMax/2
  Switch/1 -> Add/1
  Product/1 -> Delay/1, Relational Operator/1
  Add/1 -> Product/2
  Constant1/1 -> Switch/3
  Constant4/1 -> Switch/1
  u/1 -> Switch/2, Switch1/2
  Constant2/1 -> Switch1/1
  Constant3/1 -> Switch1/3
  Switch1/1 -> Product/1

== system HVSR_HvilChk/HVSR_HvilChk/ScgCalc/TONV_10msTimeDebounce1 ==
  note: Turn On Delay Time Deboune
  u : Inport
  T : Inport  Port=2
  Add : Sum
  Constant1 : Constant  Value=0  OutDataTypeStr=single
  Constant2 : Constant  OutDataTypeStr=uint8
  Constant3 : Constant  Value=0  OutDataTypeStr=uint8
  Constant4 : Constant  Value=0.01  OutDataTypeStr=single
  Delay : Delay  DelayLength=1  InitialCondition=0
  MinMax : MinMax  Inputs=2
  Product : Product  OutMin=[0]  OutMax=[65535]  OutDataTypeStr=single
  Relational Operator : RelationalOperator  Operator=>  OutDataTypeStr=boolean  RndMeth=Simplest
  Switch : Switch  Criteria=u2 ~= 0
  Switch1 : Switch  Criteria=u2 ~= 0
  y : Outport
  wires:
  Switch1/1 -> Product/1
  Constant3/1 -> Switch1/3
  Constant2/1 -> Switch1/1
  u/1 -> Switch1/2, Switch/2
  Constant4/1 -> Switch/1
  Constant1/1 -> Switch/3
  Add/1 -> Product/2
  Product/1 -> Relational Operator/1, Delay/1
  Switch/1 -> Add/1
  Delay/1 -> MinMax/2
  Relational Operator/1 -> y/1
  T/1 -> MinMax/1, Relational Operator/2
  MinMax/1 -> Add/2

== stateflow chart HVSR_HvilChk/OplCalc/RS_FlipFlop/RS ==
  state RS_FlipFlop
    (default) -> (junction 3)
    (junction 3) -> (junction 5) : [R]
    (junction 3) -> (junction 12)
    (junction 5) -> (junction 7) : {Q=boolean(0);nQ=boolean(1);}
    (junction 12) -> (junction 14) : [S]
    (junction 14) -> (junction 16) : {Q=boolean(1);nQ=boolean(0);}
    (junction 12) -> (junction 18)
    (junction 16) -> (junction 18)
    (junction 7) -> (junction 18)
    (junction 18) -> (junction 21)
  (default) -> RS_FlipFlop
  (junction 24) -> RS_FlipFlop
  (junction 25) -> (junction 24)
  RS_FlipFlop -> (junction 23)
  (junction 23) -> (junction 25)
  data: S input boolean; R input boolean; Q output boolean; nQ output boolean
